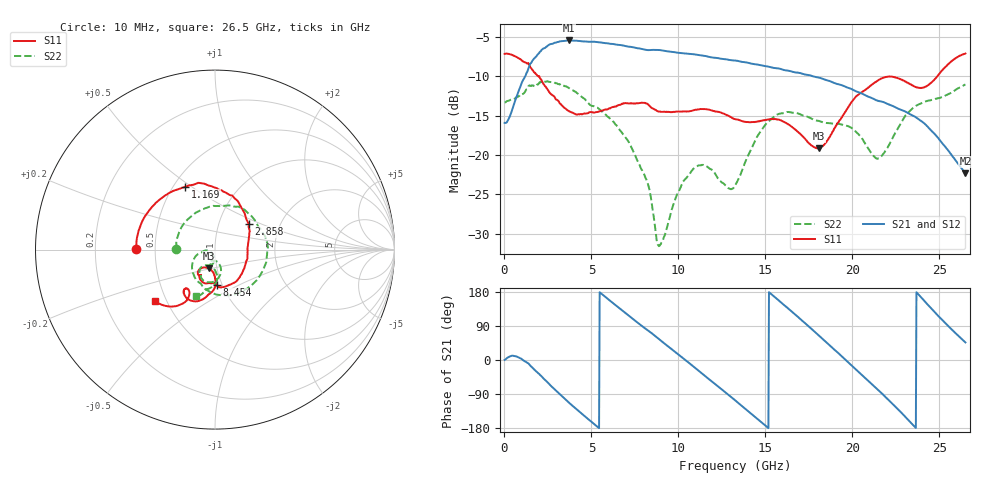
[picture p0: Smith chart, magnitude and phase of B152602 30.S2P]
!  2-Port S-parameters saved by WinCal
! VAR MeasName=S-Parameters (CALIBRATED_DATA) read from VNA (N5242A)
! VAR MeasDate=2016-1-5 16:30:37
! VAR NAME=B152602 30
! VAR FILENAME=B152602 30.S2P
! VAR DATE=2016-1-5 16:30:37
! VAR PHYS_PORTS=1,2
# Hz S DB R 50
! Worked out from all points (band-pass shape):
!   801 points, 10 MHz to 26.5 GHz, reference 50 ohm
!   highest |S21| = -5.46 dB at 3.685 GHz (marker M1); lowest = -22.3 dB at 26.5 GHz (marker M2)
!   |S21| within 3 dB of the highest: 1.474 GHz to 14.35 GHz (12.88 GHz wide, 163 % of centre)
!   lowest |S11| = -19.2 dB at 18.09 GHz (marker M3), VSWR 1.25, Z = 45.6 - j9.62 ohm
!   |S11| at or under -10 dB: 1.938 GHz to 1.988 GHz (49.77 MHz wide, 2.54 % of centre); 1.999 GHz to 24.89 GHz (22.89 GHz wide, 170 % of centre)
!   |S22| runs from -31.6 to -10.6 dB; largest |S21 - S12| = 0.0032
!   S11 on the Smith chart (normalised r, x): 10 MHz: 0.39, +0.00; 1.169 GHz: 0.57, +0.47; 2.858 GHz: 1.39, +0.42; 8.454 GHz: 0.94, -0.39; 26.5 GHz: 0.43, -0.31
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1e7  -7.16 179.4  -15.92 0.2  -15.91 0.3  -13.35 179.1
1.168938e9  -8.23 115.3  -10.10 -3.2  -10.10 -3.3  -12.04 77.1
2.029862e9  -10.18 70.2  -6.92 -38.4  -6.92 -38.4  -10.76 13.7
2.857675e9  -12.55 37.4  -5.78 -76.0  -5.78 -76.0  -10.77 -35.4
3.685488e9  -14.40 12.7  -5.46 -111.6  -5.46 -111.6  -11.47 -72.3
4.447075e9  -14.84 -4.1  -5.56 -142.1  -5.56 -142.1  -12.63 -99.0
6.036475e9  -14.07 -38.8  -5.87 157.7  -5.86 157.7  -15.31 -136.8
7.228525e9  -13.47 -63.9  -6.27 114.1  -6.26 114.1  -18.69 -160.5
8.453688e9  -14.02 -87.1  -6.65 71.1  -6.66 71.1  -25.91 -175.0
8.851038e9  -14.49 -89.6  -6.67 56.5  -6.64 56.4  -31.46 -148.3
1.077156e10  -14.39 -101.5  -7.19 -13.6  -7.16 -13.7  -22.01 -98.6
1.202984e10  -14.42 -113.5  -7.64 -60.3  -7.63 -60.6  -22.09 -113.5
1.3255e10  -15.44 -119.7  -8.01 -106.1  -8.00 -106.2  -23.89 -85.5
1.530798e10  -15.43 -120.8  -8.86 175.1  -8.83 175.1  -15.51 -86.8
1.659936e10  -16.56 -128.0  -9.45 124.4  -9.41 124.5  -14.64 -108.0
1.769208e10  -18.84 -119.3  -9.98 80.3  -9.95 80.5  -15.42 -117.6
1.808942e10  -19.17 -108.8  -10.17 64.1  -10.19 64.0  -15.68 -118.9
1.974505e10  -14.00 -89.4  -11.45 -5.3  -11.42 -5.4  -16.33 -124.6
2.136756e10  -10.71 -105.5  -13.05 -74.1  -13.00 -74.2  -20.43 -112.5
2.209604e10  -10.05 -116.1  -13.60 -106.1  -13.53 -106.3  -18.79 -90.0
2.454636e10  -10.80 -119.7  -16.91 135.7  -16.88 135.4  -13.03 -100.7
2.65e10  -7.12 -139.3  -22.35 46.4  -22.32 46.0  -11.04 -112.5
